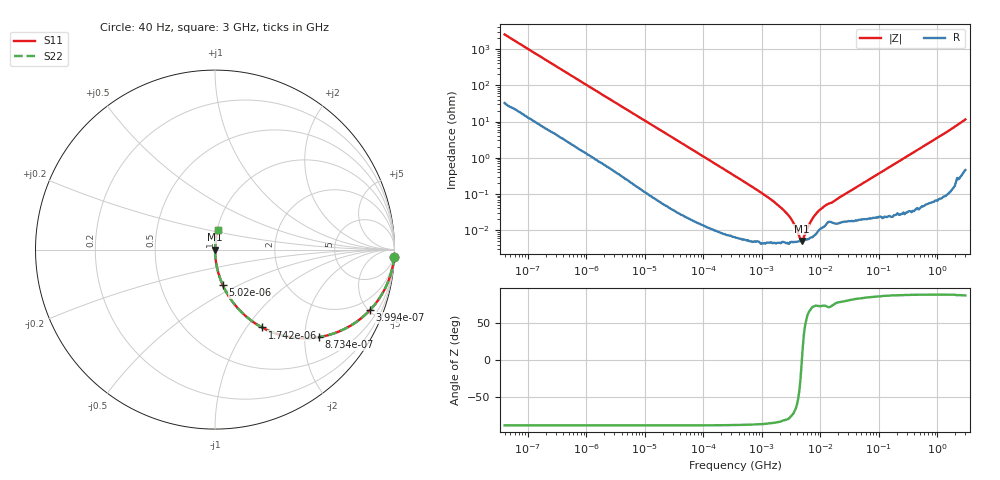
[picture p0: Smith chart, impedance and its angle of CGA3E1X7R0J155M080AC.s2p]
! S-parameter Generated by TDK Corporation
! Copyright(C) 2015 TDK Corporation.
! All Rights Reserved.
! TDK P/N: CGA3E1X7R0J155M080AC (Multilayer Ceramic Chip Capacitors)
! Property: C=1.5uF
! Size(LxWxT): 1.6x0.8x0.8mm, 0.063x0.031x0.031inches
! Model Type: s2p (Touchstone File Format Version 1.0)
! Frequency: DC=Yes Start=0.00004MHz Stop=3000MHz 396points Log-sweep
! Note: This model was converted from impedance.
! Model Generated on Jun. 23, 2015
! Hash(MD5):
! Port Assignments:
!  1 ---| |--- 2
! Applicable Conditions:
!  Temperature = 25 degC
!  DC Bias Voltage = 0 V
!  Small Signal Operation
! Terms and conditions regarding TDK Simulation Models
! (1)This simulation model is being provided solely for informational purposes. Please refer to the specifications of the products in terms of detailed characteristics of such products.
! (2)In no event shall TDK Corporation of any of its subsidiaries be liable for any loss or damage arising, directly or indirectly,
!  From any information contained in this simulation model, including, but not limited to loss or damages arising from any inaccuracies, omissions or errors in connection with such information.
! (3)Any and all copyrights on this simulation model are owned by TDK Corporation.
!  Duplication or redistribution of this simulation model without prior written permission from TDK Corporation is prohibited.
! (4)This simulation model is subject to any modification or change without any prior notice.
! (5)Neither TDK Corporation nor any of its subsidiaries shall make any warranty, express or implied,
!  Including but not limited to the correctness, implied warranties of merchantability and fitness for a particular purpose with respect to this simulation models.
! (6)The use of this simulation model shall be deemed to have consented to the terms and conditions hereof.
# MHz S MA R 50
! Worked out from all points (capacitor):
!   395 points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, 40 Hz to 3 GHz, reference 50 ohm
!   read as one part in series: C = 1.57 uF near 41.88 Hz
!   lowest |Z| = 5.01 mohm at 4.774 MHz (marker M1)
!   series resonance near 4.818 MHz, so ESL is about 690 pH
!   S11 on the Smith chart (normalised r, x): 40 Hz: 2, -51; 399.4 Hz: 1.07, -5.11; 873.4 Hz: 1.03, -2.35; 1.742 kHz: 1.01, -1.19; 5.02 kHz: 1.00, -0.42; 3 GHz: 1.01, +0.23
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4e-05  0.9987 -2.3  0.03944 87.0  0.03944 87.0  0.9987 -2.3
0.0001385867  0.9891 -7.8  0.1351 81.5  0.1351 81.5  0.9891 -7.8
0.0003994232  0.9272 -21.3  0.3627 68.0  0.3627 68.0  0.9272 -21.3
0.000834128  0.7713 -38.8  0.6269 50.5  0.6269 50.5  0.7713 -38.8
0.000873414  0.757 -40.1  0.6439 49.2  0.6439 49.2  0.757 -40.1
0.001741936  0.5071 -58.8  0.8556 30.5  0.8556 30.5  0.5071 -58.8
0.002889976  0.3367 -69.6  0.9376 19.7  0.9376 19.7  0.3367 -69.6
0.005020464  0.2033 -77.6  0.9768 11.7  0.9768 11.7  0.2033 -77.6
0.01739424  0.06097 -85.9  0.9975 3.5  0.9975 3.5  0.06097 -85.9
0.3464102  0.003129 -88.7  0.9999 0.2  0.9999 0.2  0.003129 -88.7
1.734411  0.0005515 -85.5  1 0.0  1 0.0  0.0005515 -85.5
3.013016  0.0002282 -78.3  1 0.0  1 0.0  0.0002282 -78.3
3.971241  9.801e-05 -60.8  1 0.0  1 0.0  9.801e-05 -60.8
4.773931  5.006e-05 -4.6  1 0.0  1 0.0  5.006e-05 -4.6
5.738865  9.529e-05 54.8  0.9999 -0.0  0.9999 -0.0  9.529e-05 54.8
7.22376  0.0002028 71.7  0.9999 -0.0  0.9999 -0.0  0.0002028 71.7
9.092863  0.0003277 73.4  0.9999 -0.0  0.9999 -0.0  0.0003277 73.4
12.54911  0.0004964 73.0  0.9999 -0.0  0.9999 -0.0  0.0004964 73.0
15.79611  0.0005814 73.8  0.9998 -0.0  0.9998 -0.0  0.0005814 73.8
150.6385  0.00548 87.1  0.9997 -0.3  0.9997 -0.3  0.00548 87.1
994.0817  0.03539 86.9  0.9987 -2.0  0.9987 -2.0  0.03539 86.9
3000  0.1129 81.2  0.9891 -6.5  0.9891 -6.5  0.1129 81.2
